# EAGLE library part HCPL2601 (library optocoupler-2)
HEWLETT PACKARD OPTO COUPLER
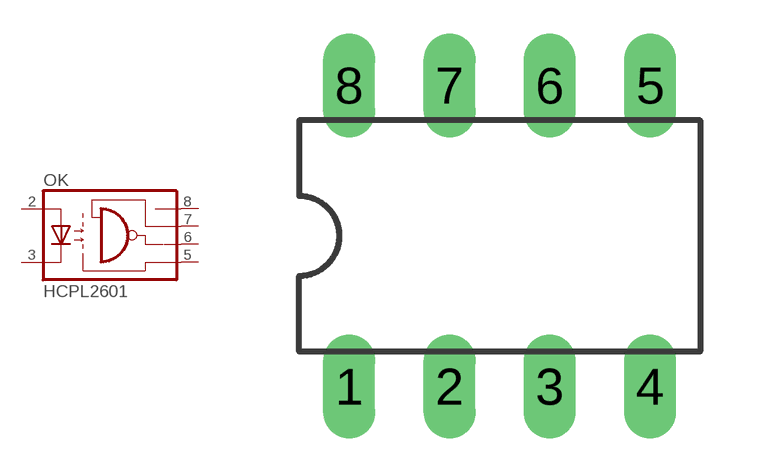
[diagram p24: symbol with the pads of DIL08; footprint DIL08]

Designator prefix OK

## HCPL2601  [DIL08]
2  A  pas
3  C  pas
5  GND  pas
6  OUT  pas
7  EN  pas
8  VCC  pas

## Footprint DIL08 (pad centres in mm)
Dual In Line Package
drill 0.813 long: 1 -3.81,-3.81; 2 -1.27,-3.81; 3 1.27,-3.81; 4 3.81,-3.81; 5 3.81,3.81; 6 1.27,3.81; 7 -1.27,3.81; 8 -3.81,3.81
